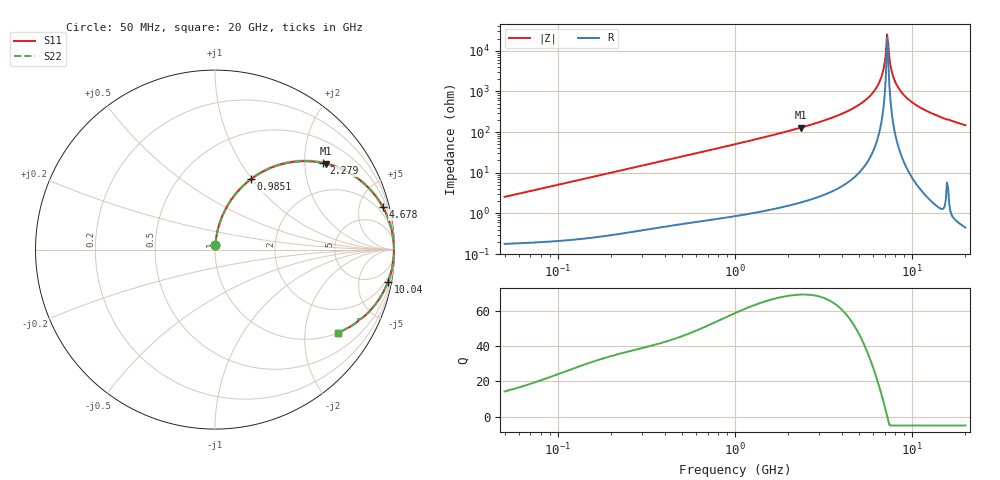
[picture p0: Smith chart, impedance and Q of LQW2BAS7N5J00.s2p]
!Murata Part Number: LQW2BAS7N5J00
!These Parameters are Measured in Series Mode Connection
!  o--[Z]--o
!Port1  Port2
!  o-------o
!Freq. Start=50[MHz] Stop=20[GHz], 401[Steps]
# Hz S RI R 50
!Freq.(Hz) S11(Real) S11(Imag) S21(Real) S21(Imag) S12(Real) S12(Imag) S22(Real) S22(Imag)
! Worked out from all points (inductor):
!   401 points, 50 MHz to 20 GHz, reference 50 ohm
!   read as one part in series: L = 8.05 nH near 51.52 MHz
!   highest Q = 69.4 at 2.349 GHz (marker M1), where L = 8.69 nH
!   self-resonance near 7.222 GHz
!   S11 on the Smith chart (normalised r, x): 50 MHz: 1.00, +0.05; 985.1 MHz: 1.02, +0.99; 2.279 GHz: 1.04, +2.47; 4.678 GHz: 1.15, +7.80; 10.04 GHz: 1, -11; 20 GHz: 1.01, -2.95
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5e7  0.00241 0.0253  0.9976 -0.0253  0.9976 -0.0253  0.00241 0.0253
1.364002e8  0.007 0.0679  0.993 -0.0679  0.993 -0.0679  0.007 0.0679
3.721004e8  0.0373 0.1778  0.9627 -0.1778  0.9627 -0.1778  0.0373 0.1778
9.85133e8  0.2 0.3915  0.8 -0.3915  0.8 -0.3915  0.2 0.3915
1e9  0.2048 0.3952  0.7952 -0.3952  0.7952 -0.3952  0.2048 0.3952
2.279204e9  0.6031 0.4821  0.3969 -0.4821  0.3969 -0.4821  0.6031 0.4821
2.348516e9  0.6202 0.4782  0.3798 -0.4782  0.3798 -0.4782  0.6202 0.4782
2.728004e9  0.7039 0.4493  0.2961 -0.4493  0.2961 -0.4493  0.7039 0.4493
4.677679e9  0.9344 0.2382  0.0656 -0.2382  0.0656 -0.2382  0.9344 0.2382
5.515528e9  0.9721 0.152  0.0279 -0.152  0.0279 -0.152  0.9721 0.152
6.217679e9  0.9888 0.0862  0.0112 -0.0862  0.0112 -0.0862  0.9888 0.0862
6.701223e9  0.9946 0.0444  0.0054 -0.0444  0.0054 -0.0444  0.9946 0.0444
6.905011e9  0.9959 0.0276  0.0041 -0.0276  0.0041 -0.0276  0.9959 0.0276
7.114996e9  0.9966 0.0107  0.00337 -0.0107  0.00337 -0.0107  0.9966 0.0107
7.331367e9  0.9968 -0.00613  0.00321 0.00613  0.00321 0.00613  0.9968 -0.00613
7.442007e9  0.9966 -0.0146  0.00335 0.0146  0.00335 0.0146  0.9966 -0.0146
7.668323e9  0.9959 -0.0314  0.00406 0.0314  0.00406 0.0314  0.9959 -0.0314
8.141811e9  0.9928 -0.0651  0.0072 0.0651  0.0072 0.0651  0.9928 -0.0651
8.907419e9  0.9838 -0.1152  0.0162 0.1152  0.0162 0.1152  0.9838 -0.1152
1.004137e10  0.9636 -0.1805  0.0364 0.1805  0.0364 0.1805  0.9636 -0.1805
1.354865e10  0.8731 -0.3298  0.1269 0.3298  0.1269 0.3298  0.8731 -0.3298
2e10  0.6845 -0.4632  0.3155 0.4632  0.3155 0.4632  0.6845 -0.4632
